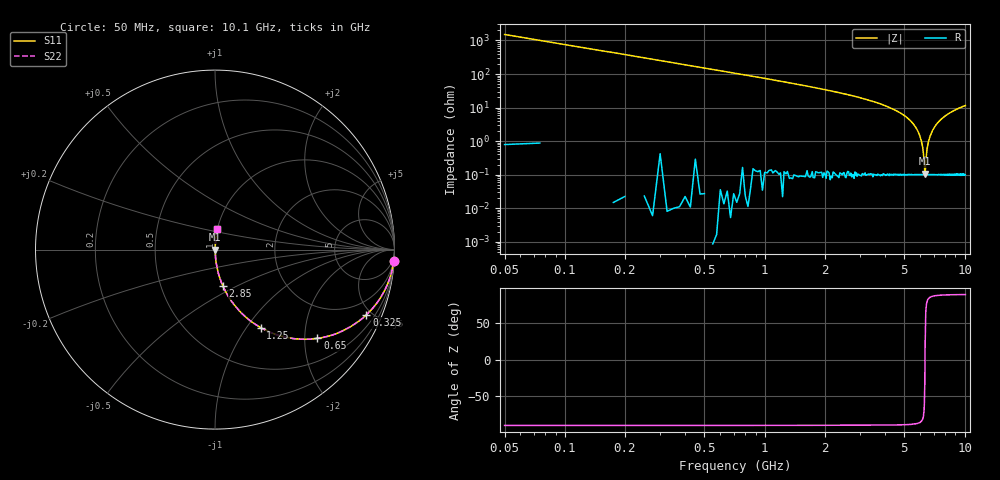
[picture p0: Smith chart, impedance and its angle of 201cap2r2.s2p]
! AVX Thin Film Operation		Date: May 2007
! Description: Accu-P® Series, Thin Film, SMD, RF Capacitor
! Part Number: 02013J2R2ABS
! 50 MHz  -  20.05 GHz
! Serial Measurements
# hz S db R 50
!	S11		S21		S12		S22
!	dB	Phase	dB	Phase	dB	Phase	dB	Phase
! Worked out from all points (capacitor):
!   400 points, 50 MHz to 10.1 GHz, reference 50 ohm
!   read as one part in series: C = 2.09 pF near 100 MHz
!   lowest |Z| = 106 mohm at 6.35 GHz (marker M1)
!   series resonance near 6.343 GHz, so ESL is about 300 pH
!   S11 on the Smith chart (normalised r, x): 50 MHz: 1, -30; 325 MHz: 1.00, -4.64; 650 MHz: 1.00, -2.31; 1.25 GHz: 1.00, -1.16; 2.85 GHz: 1.00, -0.42; 10.1 GHz: 1.00, +0.23
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5e7  -0.02 -3.8  -23.60 86.2  -23.60 86.2  -0.02 -3.8
1e8  -0.08 -7.5  -17.70 82.5  -17.70 82.5  -0.08 -7.5
1.5e8  -0.17 -11.2  -14.20 78.8  -14.20 78.8  -0.17 -11.2
3.25e8  -0.74 -23.3  -8.07 66.7  -8.07 66.7  -0.74 -23.3
6.5e8  -2.44 -40.9  -3.68 49.1  -3.68 49.1  -2.44 -40.9
1.25e9  -5.97 -59.7  -1.28 30.2  -1.28 30.2  -5.97 -59.7
1.73e9  -8.48 -67.7  -0.67 22.1  -0.67 22.1  -8.48 -67.7
2.85e9  -13.70 -77.8  -0.20 12.0  -0.20 12.0  -13.70 -77.8
3.4e9  -16.10 -80.6  -0.12 9.0  -0.12 9.0  -16.10 -80.6
5.08e9  -25.40 -85.9  -0.02 3.1  -0.02 3.1  -25.40 -85.9
5.63e9  -30.80 -86.4  -0.01 1.6  -0.01 1.6  -30.80 -86.4
6.03e9  -38.20 -84.6  -0.01 0.7  -0.01 0.7  -38.20 -84.6
6.23e9  -46.90 -77.0  -0.01 0.3  -0.01 0.3  -46.90 -77.0
6.28e9  -51.40 -68.0  -0.01 0.1  -0.01 0.1  -51.40 -68.0
6.33e9  -58.70 -30.9  -0.01 0.0  -0.01 0.0  -58.70 -30.9
6.35e9  -59.50 18.9  -0.01 -0.0  -0.01 -0.0  -59.50 18.9
6.4e9  -52.30 65.6  -0.01 -0.1  -0.01 -0.1  -52.30 65.6
6.5e9  -44.40 80.1  -0.01 -0.3  -0.01 -0.3  -44.40 80.1
6.75e9  -36.50 85.3  -0.01 -0.9  -0.01 -0.9  -36.50 85.3
7.4e9  -28.60 86.3  -0.01 -2.1  -0.01 -2.1  -28.60 86.3
8.43e9  -23.30 85.2  -0.03 -3.9  -0.03 -3.9  -23.30 85.2
1.01e10  -18.90 83.0  -0.06 -6.5  -0.06 -6.5  -18.90 83.0
